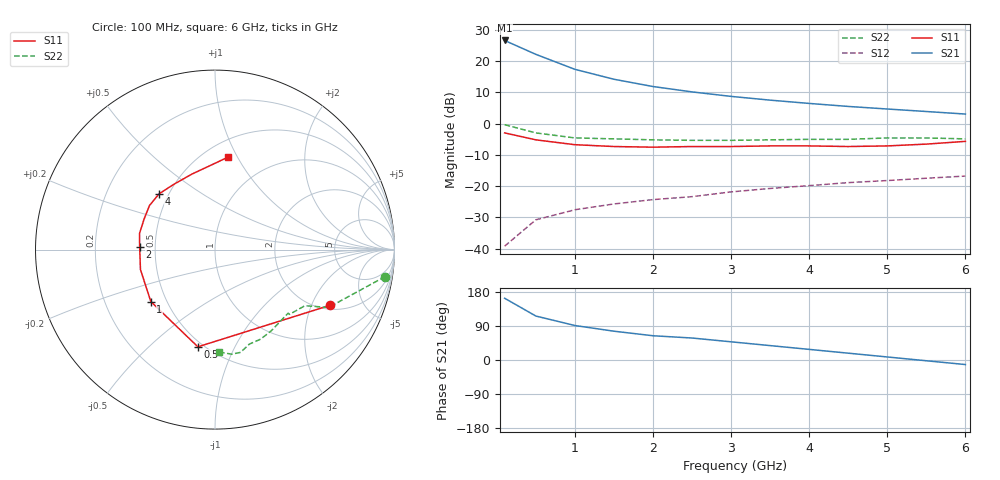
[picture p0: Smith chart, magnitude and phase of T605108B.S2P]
!AT-60510
!S-PARAMETERS at Vce=8V  Ic=10mA.  LAST UPDATED 07-21-92
# ghz s ma r 50
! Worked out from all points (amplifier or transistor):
!   13 points, 100 MHz to 6 GHz, reference 50 ohm
!   highest |S21| = 26.6 dB at 100 MHz (marker M1)
!   |S21| within 3 dB of that: start of sweep to 370 MHz
!   unconditionally stable (mu >= 1): 1.618 GHz to end of sweep
!   at 1 GHz: K = 0.82, MSG = 22.4 dB, |S12| = -27.5 dB
!   at 3 GHz: K = 1.19, MAG = 12.6 dB, |S12| = -21.8 dB
!   at 6 GHz: K = 1.03, MAG = 8.9 dB, |S12| = -16.8 dB
!   S11 on the Smith chart (normalised r, x): 100 MHz: 2.18, -2.73; 500 MHz: 0.47, -0.73; 1 GHz: 0.41, -0.30; 2 GHz: 0.41, +0.01; 4 GHz: 0.44, +0.34; 6 GHz: 0.65, +0.91
0.1  0.71 -26.0  21.3 163.0  0.011 75.0  0.96 -9.0
0.5  0.55 -100.0  12.77 116.0  0.029 51.0  0.71 -27.0
1  0.46 -141.0  7.36 91.0  0.042 44.0  0.59 -32.0
1.5  0.43 -165.0  5.11 76.0  0.052 49.0  0.57 -36.0
2  0.42 178.0  3.91 64.0  0.061 45.0  0.55 -41.0
2.5  0.43 168.0  3.21 58.0  0.068 54.0  0.54 -41.0
3  0.43 157.0  2.72 48.0  0.081 53.0  0.54 -47.0
3.5  0.44 146.0  2.37 38.0  0.092 51.0  0.55 -55.0
4  0.44 135.0  2.1 28.0  0.102 46.0  0.56 -63.0
4.5  0.43 122.0  1.88 18.0  0.114 42.0  0.56 -70.0
5  0.44 107.0  1.71 8.0  0.123 38.0  0.59 -76.0
5.5  0.47 93.0  1.56 -2.0  0.134 34.0  0.59 -81.0
6  0.52 82.0  1.42 -12.0  0.145 30.0  0.57 -88.0
